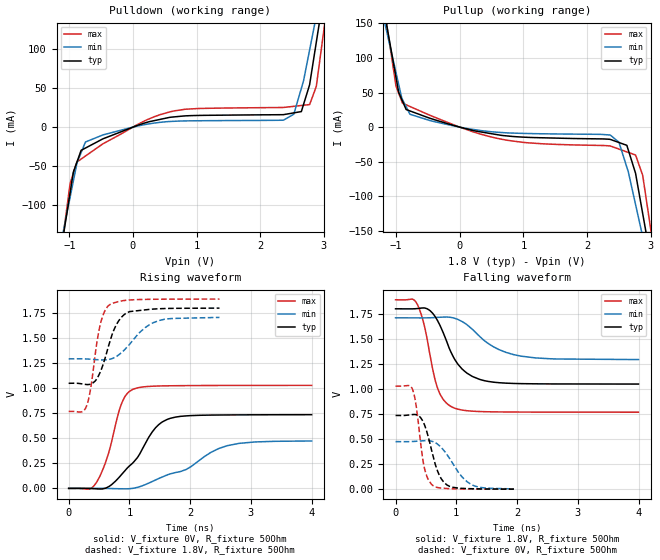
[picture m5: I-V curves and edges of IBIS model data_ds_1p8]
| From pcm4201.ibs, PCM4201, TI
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|   data_ds_1p8 Model
[Model]   data_ds_1p8
Model_type   Output
Polarity   Non-Inverting
Vmeas = 0.9
Vref = 0.9
Cref = 2pF
Rref = 50
|   typ   min   max
|   (nom PVT)   (fast PVT)   (slow PVT)
|C_comp from frequency sweep method (F=13.83MHz)
|C_comp   1.509e-12   1.305e-12   1.737e-12
|ON state : BUFFER OUTPUT TURNED HIGH
|C_comp   1.509e-12   1.305e-12   1.737e-12
|OFF state: BUFFER OUTPUT TURNED LOW
|C_comp   1.516e-12   1.344e-12   1.678e-12
|C_comp from LC tank measurement(L=1nH)
|Resonant Frequency(Hz)   7.400e+09   7.640e+09   7.170e+09
C_comp   4.630e-13   4.344e-13   4.932e-13
|ON state : BUFFER OUTPUT TURNED HIGH
|Resonant Frequency(Hz)   7.400e+09   7.640e+09   7.170e+09
|C_comp   4.630e-13   4.344e-13   4.932e-13
|OFF state: BUFFER OUTPUT TURNED LOW
|Resonant Frequency(Hz)   7.400e+09   7.680e+09   7.150e+09
|C_comp   4.630e-13   4.299e-13   4.960e-13
| Where nom  PVT is Nominal Process, 1.8V, 35C
|   Fast PVT is Strong Process,  1.89V, -10C
|   Slow PVT is Weak Process,   1.71V, 80C
[Voltage Range]   1.8   1.71   1.89
|Ambient Temperature   25   70   -10
|Junction Temperature
[Temperature Range]   35   80   -10
[Pullup Reference]   1.8   1.71   1.89
[Pulldown Reference]   0   0   0
[Power Clamp Reference]   1.8   1.71   1.89
[GND Clamp Reference]   0   0   0
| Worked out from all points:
|   slope of the pulldown table from 0 to 0.27 V, typ, clamps not added: 37.4 ohm
|   slope of the pullup table from 0 to 0.27 V, typ, clamps not added: 45.3 ohm
|   falling waveform, V_fixture 1.8V, R_fixture 50Ohm: 20-80 % time 377ps typ, 566ps min, 242ps max; typ from 1.8 V to 1.05 V
|   rising waveform, V_fixture 0V, R_fixture 50Ohm: 20-80 % time 524ps typ, 937ps min, 283ps max; typ from 0 V to 0.736 V
|   rising waveform, V_fixture 1.8V, R_fixture 50Ohm: 20-80 % time 255ps typ, 400ps min, 172ps max; typ from 1.05 V to 1.8 V
|   falling waveform, V_fixture 0V, R_fixture 50Ohm: 20-80 % time 208ps typ, 333ps min, 136ps max; typ from 0.736 V to 0.001 V
[Pulldown]
|   Voltage   I(typ)   I(min)   I(max)
-1.8V     -507.1mA   -421.2mA   -630.4mA
-1.238V   -213.8mA   -192.2mA   -227.7mA
-988.5mV  -85.08mA   -90.63mA   -73.25mA
-813.6mV  -29.73mA   -32.72mA   -40.9mA
-471.6mV  -15.02mA   -10.01mA   -21.4mA
653.9mV   13.19mA    7.521mA    20.87mA
2.365V    15.98mA    8.874mA    25.2mA
2.529V    18.28mA    16.57mA    26.68mA
2.648V    19.95mA    49.71mA    27.75mA
2.884V    109.4mA    143.1mA    52.93mA
3.103V    222.9mA    234.2mA    186mA
3.6V      486.1mA    440.5mA    540.3mA
[Pullup]
|   Voltage   I(typ)   I(min)   I(max)
-1.8V     486.4mA    402.6mA    606.4mA
-1.246V   197.3mA    177.6mA    208.7mA
-1.002V   71.71mA    78.73mA    59.22mA
-783.2mV  23.41mA    18.65mA    29.85mA
655.8mV   -11.9mA    -7.77mA    -17.45mA
2.365V    -17.68mA   -11.38mA   -27.18mA
2.502V    -22.19mA   -21.76mA   -31.68mA
2.626V    -26.29mA   -57.91mA   -35.78mA
2.763V    -66.63mA   -111.7mA   -40.28mA
2.875V    -124.5mA   -158mA     -69.36mA
3.103V    -243.3mA   -252.9mA   -210.3mA
3.6V      -506.9mA   -458.9mA   -564.5mA
[Ramp]
R_load = 50
|   typ   min   max
dV/dt_r   0.441368/5.23045e-10   0.283939/9.31949e-10   0.616949/2.82498e-10
dV/dt_f   0.450474/3.76601e-10   0.249915/5.60403e-10   0.672853/2.41317e-10
[Falling Waveform]
V_fixture = 1.8V
V_fixture_min = 1.71V
V_fixture_max = 1.89V
R_fixture = 50Ohm
|   Time   V(typ)   V(min)   V(max)
0s        1.8V       1.71V      1.89V
356ps     1.802V     1.71V      1.847V
470ps     1.809V     1.71V      1.641V
688ps     1.686V     1.714V     1.015V
792ps     1.551V     1.717V     889.9mV
938ps     1.336V     1.711V     817.7mV
1.272ns   1.123V     1.591V     778.5mV
1.606ns   1.069V     1.423V     772.1mV
1.954ns   1.055V     1.341V     770.3mV
3.998ns   1.049V     1.293V     768.6mV
[Rising Waveform]
V_fixture = 0V
V_fixture_min = 0V
V_fixture_max = 0V
R_fixture = 50Ohm
|   Time   V(typ)   V(min)   V(max)
0s        642.3pV    1.279nV    373.2pV
340ps     -448uV     319.3uV    -5.828mV
456ps     -4.46mV    254.4uV    57.89mV
658ps     17.07mV    -1.036mV   354mV
872ps     139.3mV    -4.061mV   848.9mV
1.056ns   254.6mV    532uV      988.2mV
1.428ns   604.1mV    83.67mV    1.021V
1.674ns   699.5mV    145.1mV    1.024V
2.612ns   733.2mV    426.6mV    1.028V
3.998ns   735.6mV    473.2mV    1.028V
[Rising Waveform]
V_fixture = 1.8V
V_fixture_min = 1.71V
V_fixture_max = 1.89V
R_fixture = 50Ohm
|   Time   V(typ)   V(min)   V(max)
0s        1.049V     1.293V     768.5mV
216ps     1.043V     1.293V     764.6mV
298ps     1.037V     1.292V     828.7mV
360ps     1.04V      1.289V     990.9mV
518ps     1.159V     1.283V     1.632V
654ps     1.417V     1.286V     1.823V
814ps     1.664V     1.329V     1.864V
994ps     1.763V     1.432V     1.88V
1.49ns    1.793V     1.676V     1.888V
2.482ns   1.8V       1.707V     1.89V
[Falling Waveform]
V_fixture = 0V
V_fixture_min = 0V
V_fixture_max = 0V
R_fixture = 50Ohm
|   Time   V(typ)   V(min)   V(max)
0s        736.1mV    475.1mV    1.028V
282ps     745.1mV    476.4mV    992.3mV
340ps     743.7mV    478.5mV    828mV
466ps     657.4mV    484.2mV    237.2mV
592ps     391.6mV    479.7mV    49.01mV
726ps     133.3mV    431.9mV    13.7mV
888ps     29.41mV    309mV      5.97mV
1.078ns   9.612mV    135.3mV    3.127mV
1.248ns   5.172mV    46.84mV    2.13mV
1.948ns   1.366mV    3.323mV    776.5uV
